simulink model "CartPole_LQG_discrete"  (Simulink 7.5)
settings: Solver=ode45  StartTime=0.0  StopTime=10.0  RelTol=1e-3
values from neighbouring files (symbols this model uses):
  Cmis = [1 0 0 0;0 0 1 0]    [Esercitazione09.m]
  d_theta = 0.0001    [Esercitazione09.m]
  d_w = 0.05    [Esercitazione09.m]
  d_x = 0.001    [Esercitazione09.m]
  g = 9.81    [Esercitazione09.m]
  K = lqrd(A,B,Q,R,Ts)    [Esercitazione09.m]
  L = 1    [Esercitazione09.m]
  Lobs = -LKalman    [Esercitazione09.m]
  m = 0.1    [Esercitazione09.m]
  M = 1    [Esercitazione09.m]
  Ts = 0.01    [Esercitazione09.m]
  ue = 0    [Esercitazione09.m]
  X0 = [1 0 0.55 0]'    [Esercitazione09.m]
  Xe = [1 0 0 0]'    [Esercitazione09.m]
undefined symbols (not defined in the file or in its folder): Az, Bz, Cz

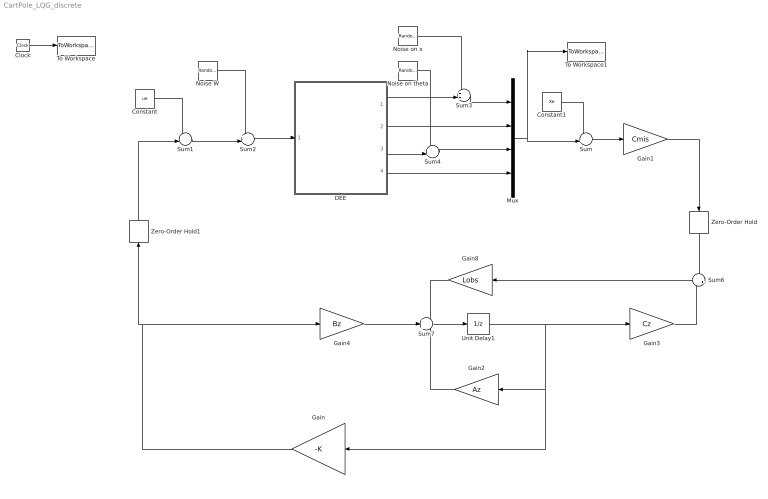
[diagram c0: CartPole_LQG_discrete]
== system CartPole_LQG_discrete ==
  Clock : Clock
  Constant : Constant  Value=ue  OutDataType=fixdt(1, 16)  OutScaling=2^0
  Constant1 : Constant  Value=Xe  OutDataType=fixdt(1, 16)  OutScaling=2^0
  DEE : Subsystem
  Gain : Gain  Gain=-K  Multiplication=Matrix(K*u)  ParameterDataType=fixdt(1, 16)  ParameterScaling=2^0  OutDataType=fixdt(1, 16)  OutScaling=2^0
  Gain1 : Gain  Gain=Cmis  Multiplication=Matrix(K*u)  ParameterDataType=sfix(16)  ParameterScaling=2^0  OutDataType=sfix(16)  OutScaling=2^0
  Gain2 : Gain  Gain=Az  Multiplication=Matrix(K*u)  ParameterDataType=sfix(16)  ParameterScaling=2^0  OutDataType=sfix(16)  OutScaling=2^0
  Gain3 : Gain  Gain=Cz  Multiplication=Matrix(K*u)  ParameterDataType=sfix(16)  ParameterScaling=2^0  OutDataType=sfix(16)  OutScaling=2^0
  Gain4 : Gain  Gain=Bz  Multiplication=Matrix(K*u)  ParameterDataType=sfix(16)  ParameterScaling=2^0  OutDataType=sfix(16)  OutScaling=2^0
  Gain8 : Gain  Gain=Lobs  Multiplication=Matrix(K*u)  ParameterDataType=sfix(16)  ParameterScaling=2^0  OutDataType=sfix(16)  OutScaling=2^0
  Mux : Mux
  Noise W : RandomNumber  Variance=d_w  SampleTime=0
  Noise on theta : RandomNumber  Variance=d_theta  SampleTime=0
  Noise on x : RandomNumber  Variance=d_x  SampleTime=0
  Sum : Sum  Inputs=-+|  OutDataType=fixdt(1, 16)  OutScaling=2^0
  Sum{1..4} (4 alike) : Sum  Inputs=++|  OutDataType=fixdt(1, 16)  OutScaling=2^0
  Sum6 : Sum  Inputs=-+  OutDataType=sfix(16)  OutScaling=2^0
  Sum7 : Sum  Inputs=+++  OutDataType=sfix(16)  OutScaling=2^0
  To Workspace : ToWorkspace  VariableName=time  SampleTime=-1  SaveFormat=Array
  To Workspace1 : ToWorkspace  VariableName=X  SampleTime=-1  SaveFormat=Array
  Unit Delay1 : UnitDelay  X0=[0 0 0 0]'  SampleTime=Ts
  Zero-Order Hold : ZeroOrderHold  SampleTime=Ts
  Zero-Order Hold1 : ZeroOrderHold  SampleTime=Ts
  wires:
  DEE/2(Port2) -> Mux/2
  DEE/4(Port4) -> Mux/4
  Clock/1 -> To Workspace/1
  Mux/1 -> Sum/2, To Workspace1/1
  Constant/1 -> Sum1/1
  Constant1/1 -> Sum/1
  Sum2/1 -> DEE/1(SysInport1)
  Sum1/1 -> Sum2/2
  Noise W/1 -> Sum2/1
  Noise on x/1 -> Sum3/1
  Sum3/1 -> Mux/1
  DEE/1(Port1) -> Sum3/2
  Noise on theta/1 -> Sum4/1
  DEE/3(Port3) -> Sum4/2
  Sum4/1 -> Mux/3
  Gain1/1 -> Zero-Order Hold/1
  Sum/1 -> Gain1/1
  Zero-Order Hold1/1 -> Sum1/2
  Gain/1 -> Gain4/1, Zero-Order Hold1/1
  Unit Delay1/1 -> Gain3/1, Gain2/1, Gain/1
  Sum7/1 -> Unit Delay1/1
  Gain3/1 -> Sum6/2
  Sum6/1 -> Gain8/1
  Gain8/1 -> Sum7/1
  Gain2/1 -> Sum7/3
  Gain4/1 -> Sum7/2
  Zero-Order Hold/1 -> Sum6/1

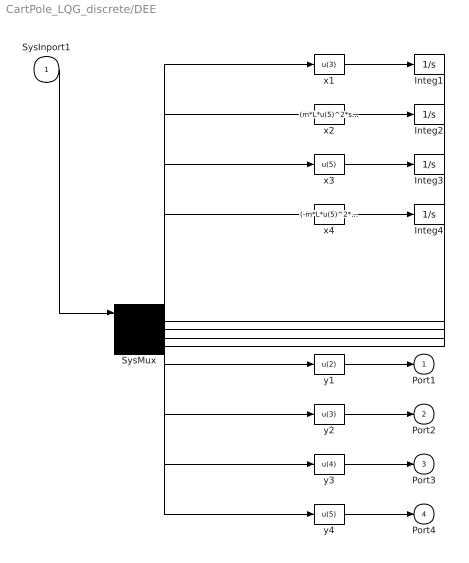
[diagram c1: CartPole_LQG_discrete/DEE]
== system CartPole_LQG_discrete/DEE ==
  SysInport1 : Inport
  Integ1 : Integrator  InitialCondition=X0(1)
  Integ2 : Integrator  InitialCondition=X0(2)
  Integ3 : Integrator  InitialCondition=X0(3)
  Integ4 : Integrator  InitialCondition=X0(4)
  SysMux : Mux  Inputs=5
  x1 : Fcn  Expr=u(3)
  x2 : Fcn  Expr=(m*L*u(5)^2*sin(u(4)) - m*g*sin(u(4))*cos(u(4))+ u)/(M+m*sin(u(4))^2)
  x3 : Fcn  Expr=u(5)
  x4 : Fcn  Expr=(-m*L*u(5)^2*sin(u(4))*cos(u(4))+(M+m)*g*sin(u(4))-u*cos(u(4)))/((M+m*sin(u(4))^2)*L)
  y1 : Fcn  Expr=u(2)
  y2 : Fcn  Expr=u(3)
  y3 : Fcn  Expr=u(4)
  y4 : Fcn  Expr=u(5)
  Port1 : Outport
  Port2 : Outport  Port=2
  Port3 : Outport  Port=3
  Port4 : Outport  Port=4
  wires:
  SysInport1/1 -> SysMux/1
  SysMux/1 -> x1/1, x2/1, x3/1, x4/1, y1/1, y2/1, y3/1, y4/1
  x1/1 -> Integ1/1
  Integ1/1 -> SysMux/2
  x2/1 -> Integ2/1
  Integ2/1 -> SysMux/3
  x3/1 -> Integ3/1
  Integ3/1 -> SysMux/4
  x4/1 -> Integ4/1
  Integ4/1 -> SysMux/5
  y1/1 -> Port1/1
  y2/1 -> Port2/1
  y3/1 -> Port3/1
  y4/1 -> Port4/1
